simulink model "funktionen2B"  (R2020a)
settings: Solver=ode45  StartTime=0.0  StopTime=10.0  MaxStep=1e-2  RelTol=1e-3  EnableMultiTasking=on
libraries: simulink x1

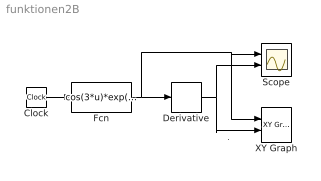
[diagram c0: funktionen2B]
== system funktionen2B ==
  note: .
  Clock : Clock
  Derivative : Derivative
  Fcn : Fcn  Expr=cos(3*u)*exp(-0.3*u)
  Scope : Scope  NumInputPorts=2
  XY Graph : simulink/Sinks/XY Graph  xmin=-1  xmax=1  ymin=-2.7  ymax=2.7  st=-1
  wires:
  Derivative/1 -> Scope/2, XY Graph/2
  Fcn/1 -> Derivative/1, Scope/1, XY Graph/1
  Clock/1 -> Fcn/1
